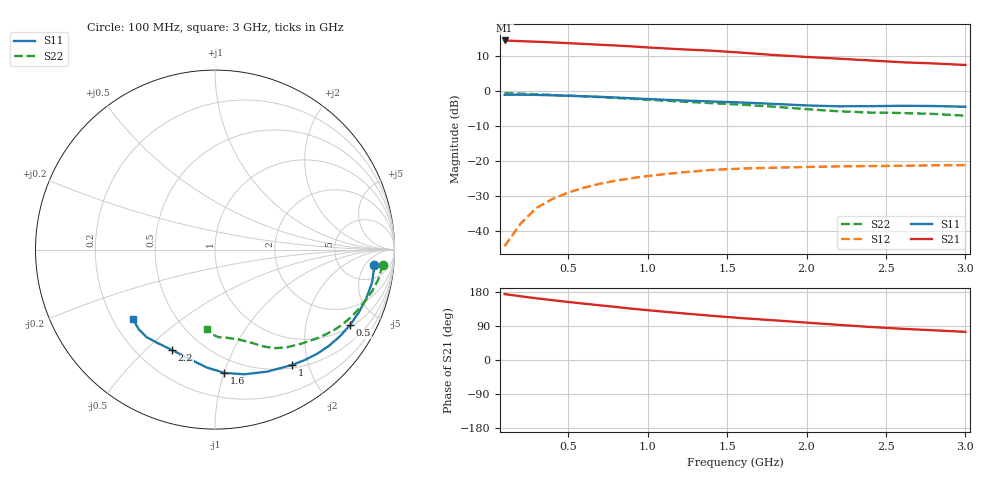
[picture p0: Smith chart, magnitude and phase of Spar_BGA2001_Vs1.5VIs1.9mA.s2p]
! Filename: 1_5VG1.001
! Title: BGA2001 X0297-20 HFE=80
! Bias: Vce=1.5V,Ic=1.9mA
! Company: NXP Semiconductors NL
! User: Quality&Reliability T&D
! Measure time: 23 Oct 1998 / 09:09:17
#  MHz  S  MA  R 50
! Freq  S11  S21  S12  S22  :
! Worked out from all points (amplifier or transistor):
!   20 points, 100 MHz to 3 GHz, reference 50 ohm
!   highest |S21| = 14.5 dB at 100 MHz (marker M1)
!   |S21| within 3 dB of that: start of sweep to 1.428 GHz
!   unconditionally stable (mu >= 1): 2.88 GHz to end of sweep
!   at 400 MHz: K = 0.17, MSG = 22.4 dB, |S12| = -30.8 dB
!   at 1.2 GHz: K = 0.37, MSG = 17.6 dB, |S12| = -23.3 dB
!   at 3 GHz: K = 1.08, MAG = 12.6 dB, |S12| = -21.1 dB
!   S11 on the Smith chart (normalised r, x): 100 MHz: 10, -9; 500 MHz: 1.08, -3.52; 1 GHz: 0.55, -1.74; 1.6 GHz: 0.38, -1.00; 2.2 GHz: 0.34, -0.61; 3 GHz: 0.28, -0.34
100  0.8923 -5.6  5.321 173.9  0.006081 57.1  0.9379 -5.2
200  0.8943 -11.6  5.2 168.2  0.01272 82.8  0.9255 -10.2
300  0.8861 -17.7  5.104 162.9  0.02138 79.5  0.9055 -14.9
400  0.8743 -23.6  4.993 157.9  0.02871 75.4  0.8839 -19.1
500  0.8616 -29.3  4.868 153.2  0.03554 71.8  0.8634 -23.0
600  0.8469 -34.9  4.749 148.7  0.04177 68.3  0.8434 -26.8
700  0.8308 -40.3  4.619 144.3  0.04748 65.1  0.8241 -30.4
800  0.8125 -45.6  4.507 140.0  0.05263 62.0  0.8016 -33.9
900  0.7925 -51.0  4.375 135.4  0.05709 59.0  0.7784 -37.2
1000  0.7733 -56.2  4.228 131.5  0.06125 56.4  0.7558 -40.6
1200  0.7397 -66.8  3.991 123.8  0.06858 51.5  0.712 -47.4
1400  0.7135 -76.8  3.803 116.8  0.07473 47.1  0.6758 -53.7
1600  0.6885 -85.8  3.552 110.2  0.07846 44.0  0.6405 -59.1
1800  0.6578 -94.1  3.287 104.7  0.08059 42.2  0.6002 -63.8
2000  0.6259 -103.2  3.091 98.6  0.08254 39.3  0.5544 -69.0
2200  0.6088 -113.0  2.923 92.8  0.08413 36.7  0.5166 -75.5
2400  0.611 -121.6  2.757 87.2  0.08506 35.2  0.4956 -82.4
2600  0.6192 -128.2  2.595 82.5  0.08573 35.5  0.488 -87.8
2800  0.6141 -133.8  2.496 78.4  0.08726 34.9  0.4738 -91.5
3000  0.5996 -139.9  2.374 74.3  0.08771 35.1  0.4462 -95.4
